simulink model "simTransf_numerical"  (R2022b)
settings: Solver=ode15s  StartTime=0.0  StopTime=tsim  FixedStep=0.1  MaxStep=1  RelTol=1e-5
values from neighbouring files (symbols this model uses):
  C = Fc*cpc/(Fh*cph)    [calcblock.m]    (also in calcblock2.m; calcblock3.m; calcv0.m; eNTU.m = m.c*cp.c/(m.h*cp.h))
  d_tstep = [500; 50000; 70000; 130000; 50000; 50000]    [runTransf.m]    (also in runTransfOL.m = [500 5000 7000 13000]; Main.m = [1000; 1000;2000]; Main_OL.m = 300; runTestCalcBlk.m = 300)
  dFc = -0.5    [runTransfOL.m]    (also in Main_OL.m = dist(i); Main.m = 0)
  dFh = 2    [runTransf.m]    (also in runTransfOL.m = 0; Main.m = 0;0.2*Fh)
  dTcin = 0    [runTransf.m]    (also in runTransfOL.m; Main.m = 2)
  dThin = 0    [runTransf.m]    (also in runTransfOL.m; Main.m = 0;2)
  dv2 = -0.3910    (= -0.391)    [FcOL.m]    (also in runTransfOL.m = -1)
  Fc0 = 5    [runTransf.m]    (also in runTransfOL.m; Main.m; Main_OL.m; runTestCalcBlk.m)
  Fh = d(1)    [calcblock.m]    (also in calcblock2.m; calcblock3.m; calcblockv2.m; calcv0.m)
  Kc = 1/kM(i)*tau(i)/(tauCM(i)+theta(i))    [runTransf.m]    (also in runTransfOL.m; Main.m = 1/k*tau/(tauC+theta))
  KI = 1/kS(i)*1/tauCS(i)    [runTransf.m]    (also in runTransfOL.m; Main.m = Kp/tauIv; Main_OL.m = 1)
  nd = size(d0,1)    [runTransf.m]    (also in runTransfOL.m = size(d0,2); Main.m = size(d0,2); Main_OL.m = size(d0,2); runTestCalcBlk.m = size(d0,2))
  np = size(p,2)    [runTransf.m]    (also in runTransfOL.m; runH2Psim.m = length(param); Main.m; Main_OL.m)
  nu = 1    [runTransf.m]    (also in runTransfOL.m; runH2Psim.m = length(u0); Main.m; Main_OL.m)
  nx = size(x0,1)    [runTransf.m]    (also in runTransfOL.m; H2P_Turbine_driven.m = param(end); runTD.m = length(x0); H2P_Boiler_driven.m = param(end))
  p = [U;A;Fc(i);Fh;cpc;cph;Tcin;Thin]    [NonlinearMap.m]    (also in runTransf.m = [N, Fc0, rhoc, rhoh, U0, A,cpc,cph]; runTransfOL.m = [N, Fc0, rhoc, rhoh, U0, A,cpc,cph]; Main.m = [N, Fc0, rhoc, rhoh,U,A,cpc,cph]; Main_OL.m = [N, Fc0, rhoc, rhoh,U,A,cpc,cph])
  pi_ff = 0    [runTransfOL.m]    (also in Main.m; Main_OL.m)
  Tcin = d(2)    [calcblock.m]    (also in calcblock2.m; calcblock3.m; calcblockv2.m; calcv0.m)
  Thin = d(3)    [calcblock.m]    (also in calcblock2.m; calcblock3.m; calcblockv2.m; calcv0.m)
  Thsp = Thsp0    [runTransf.m]    (also in runTransfOL.m; Main.m = Thsp0+dThsp; Main_OL.m = Thsp0+dThsp; runTestCalcBlk.m = Thsp0+dThsp)
  Thsp0 = x0(end-1);  2.971202611676064e+02    [runTransf.m]    (also in runTransfOL.m = x0(end);  2.971202611676064e+02; Main.m = Thend(end); Main_OL.m = 297.120261168; runTestCalcBlk.m = Thend(end))
  tstep = 10000    [runTransf.m]    (also in runTransfOL.m = 100; Main_OL.m = 100; Main.m = 100)
  v00 = calcv0(0,Fc0,p,d0)    [runTransf.m]    (also in runTransfOL.m)
  v20 = v00    [runTransfOL.m]
  vf = v00    [runTransfOL.m]    (also in Main.m = v0+dThsp; runTransf.m = 0)
  x0 = [Tcend(1:N)'; Thend(1:N)';Thin]    [runTransf.m]    (also in runTransfOL.m = [Tcend(1:N)'; Thend(1:N)']; runTD.m = [TE0;TD0;TSh0;MD0; MSh0;w0;TA0;0;0;0;0;0;0;0;0;0]; runBD.m = [TE0;TD0;TSh0;MD0; MSh0;w0;TA0;0;0;0;0;0;0;0;0;0]; runFP.m = [TE0;TD0;TSh0;MD0; MSh0;w0;TA0;0;0;0;0;0;0;0])
undefined symbols (not defined in the file or in its folder): calcblockv2, calcv0, calcv2, HEXode

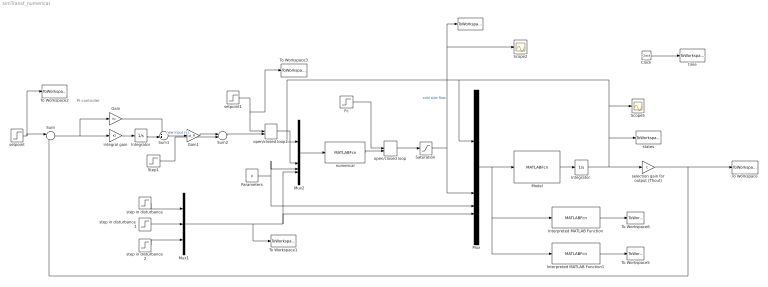
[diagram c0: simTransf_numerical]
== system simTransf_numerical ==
  note: PI-controller
  " " : ToWorkspace  VariableName=u  SampleTime=-1
  Clock : Clock
  Fc : Step  Time=tstep  Before=Fc0  After=Fc0+dFc  SampleTime=0
  Gain : Gain  Gain=Kc
  Gain1 : Gain  Gain=pi_ff  Multiplication=Matrix(K*u)
  Integrator : Integrator
  "Integrator " : Integrator  InitialCondition=x0
  Interpreted MATLAB Function : MATLABFcn  MATLABFcn=calcv0(u(1:nx),u(nx+1:nx+nu),u(nx+nu+1:nx+nu+np),u(nx+nu+np+1:nx+nu+np+nd))  OutputDimensions=1
  Interpreted MATLAB Function1 : MATLABFcn  MATLABFcn=calcv2(u(1:nx),u(nx+1:nx+nu),u(nx+nu+1:nx+nu+np),u(nx+nu+np+1:nx+nu+np+nd))  OutputDimensions=1
  Model : MATLABFcn  MATLABFcn=HEXode(u(1:nx),u(nx+1:nx+nu),u(nx+nu+1:nx+nu+np),u(nx+nu+np+1:nx+nu+np+nd))  OutputDimensions=nx  Output1D=off
  Mux : Mux
  Mux1 : Mux  Inputs=3
  Mux2 : Mux
  Parameters : Constant  Value=p
  "Saturation " : Saturate  UpperLimit=inf  LowerLimit=0
  Scope2 : Scope
  Scope5 : Scope
  Step1 : Step  Time=tstep  Before=v00  After=vf  SampleTime=0
  Sum : Sum  Inputs=|+-
  Sum1 : Sum  Inputs=++|
  Sum2 : Sum  Inputs=|++
  To Workspace : ToWorkspace  VariableName=Thout  SampleTime=-1
  To Workspace1 : ToWorkspace  VariableName=d  SampleTime=-1
  To Workspace2 : ToWorkspace  VariableName=Tsp  SampleTime=-1
  To Workspace3 : ToWorkspace  VariableName=vsp  SampleTime=-1
  To Workspace5 : ToWorkspace  VariableName=v2  SampleTime=-1
  To Workspace6 : ToWorkspace  VariableName=v0  SampleTime=-1
  integral gain : Gain  Gain=KI  Multiplication=Matrix(K*u)
  numerical : MATLABFcn  MATLABFcn=calcblockv2(u(1:nx),u(nx+1:nx+nu),u(nx+nu+1:nx+nu+np),u(nx+nu+np+1:nx+nu+np+nd))
  open/closed loop : ManualSwitch
  open/closed loop1 : ManualSwitch
  selection gain for output (Thout) : Gain  Gain=C  Multiplication=Matrix(K*u)
  setpoint : Step  Time=tstep  Before=Thsp0  After=Thsp  SampleTime=0
  setpoint1 : Step  Time=tstep  Before=v20  After=v20+dv2  SampleTime=0
  states : ToWorkspace  VariableName=y  SampleTime=-1
  step in disturbance : Step  Time=d_tstep(1)  Before=Fh  After=Fh+dFh  SampleTime=0
  step in disturbance1 : Step  Time=d_tstep(2)  Before=Tcin  After=Tcin+dTcin  SampleTime=0
  step in disturbance2 : Step  Time=d_tstep(3)  Before=Thin  After=Thin+dThin  SampleTime=0
  time : ToWorkspace  VariableName=t  SampleTime=-1
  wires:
  Model/1 -> "Integrator "/1
  "Integrator "/1 -> selection gain for output (Thout)/1, states/1, Mux2/1, Mux/1, Scope5/1
  Mux/1 -> Interpreted MATLAB Function1/1, Interpreted MATLAB Function/1, Model/1
  Clock/1 -> time/1
  Parameters/1 -> Mux/3, Mux2/3
  "Saturation "/1 -> Mux/2, Scope2/1, " "/1  "cold side flow"
  numerical/1 -> open/closed loop/2
  setpoint/1 -> To Workspace2/1, Sum/1
  Sum/1 -> Gain/1, integral gain/1
  integral gain/1 -> Integrator/1
  Sum1/1 -> Gain1/1  "new input (v)"
  selection gain for output (Thout)/1 -> Sum/2, To Workspace/1
  Mux2/1 -> numerical/1
  Step1/1 -> Sum2/2
  open/closed loop/1 -> "Saturation "/1
  Fc/1 -> open/closed loop/1
  Integrator/1 -> Sum1/2
  open/closed loop1/1 -> Mux2/2
  setpoint1/1 -> To Workspace3/1, open/closed loop1/1
  Gain/1 -> Sum1/1
  Gain1/1 -> Sum2/1
  Sum2/1 -> open/closed loop1/2
  Mux1/1 -> Mux2/4, Mux/4, To Workspace1/1
  step in disturbance/1 -> Mux1/1
  step in disturbance1/1 -> Mux1/2
  step in disturbance2/1 -> Mux1/3
  Interpreted MATLAB Function1/1 -> To Workspace5/1
  Interpreted MATLAB Function/1 -> To Workspace6/1
